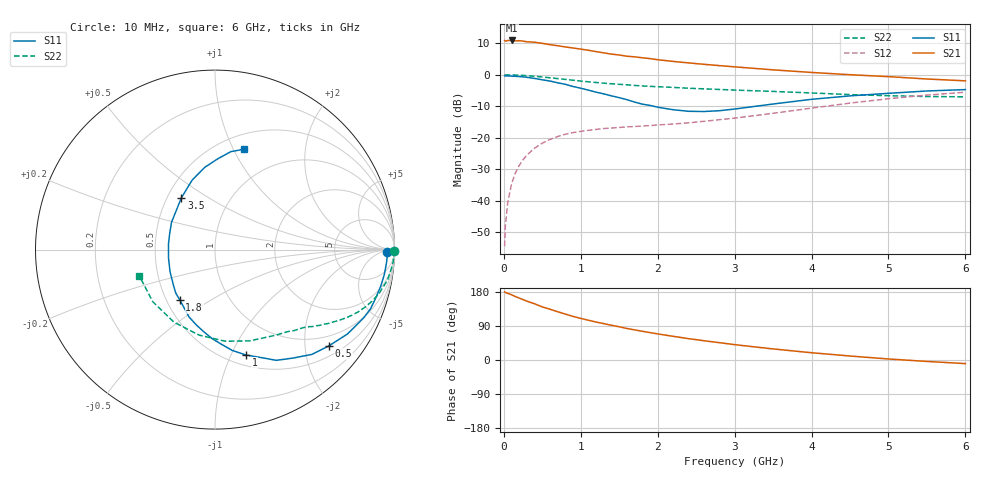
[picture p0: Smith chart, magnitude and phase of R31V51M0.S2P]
! SIEMENS Small Signal Semiconductors
! BFR181
! Si NPN RF Bipolar Junction Transistor in SOT23
! VCE = 1.5 V  IC = 1 mA
! Common Emitter S-Parameters:  May  1996
# GHz  S  MA  R  50
!  f  S11  S21  S12  S22
! GHz  MAG  ANG  MAG  ANG  MAG  ANG  MAG  ANG
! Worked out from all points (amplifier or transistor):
!   36 points, 10 MHz to 6 GHz, reference 50 ohm
!   highest |S21| = 10.9 dB at 100 MHz (marker M1)
!   |S21| within 3 dB of that: start of sweep to 1.068 GHz
!   unconditionally stable (mu >= 1): 1.968 GHz to 3.727 GHz
!   at 250 MHz: K = 0.16, MSG = 18.8 dB, |S12| = -27.0 dB
!   at 1.4 GHz: K = 0.78, MSG = 11.7 dB, |S12| = -16.9 dB
!   at 6 GHz: K = 0.89, MSG = 1.8 dB, |S12| = -5.5 dB
!   S11 on the Smith chart (normalised r, x): 10 MHz: 42, -16; 500 MHz: 0.73, -2.54; 1 GHz: 0.61, -1.14; 1.8 GHz: 0.59, -0.37; 3.5 GHz: 0.59, +0.39; 6 GHz: 0.65, +1.10
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0.01  0.9588 -0.9  3.478 179.5  0.0019 89.5  0.9987 -0.4
0.02  0.9605 -1.6  3.413 178.2  0.004 93.6  0.9934 -0.8
0.05  0.9586 -4.4  3.503 176.0  0.0092 87.2  0.997 -1.9
0.1  0.9534 -8.4  3.506 172.2  0.0185 84.1  0.9945 -4.0
0.15  0.9456 -12.5  3.454 167.3  0.0276 81.4  0.989 -5.9
0.2  0.9358 -16.5  3.476 163.4  0.0363 78.9  0.9825 -7.9
0.3  0.9111 -24.7  3.341 155.3  0.0533 74.4  0.9668 -11.4
0.4  0.8751 -32.5  3.288 148.3  0.0683 69.6  0.9466 -14.9
0.5  0.8304 -40.3  3.156 140.1  0.0821 65.1  0.9218 -18.1
0.7  0.7449 -54.2  2.894 127.4  0.1047 57.5  0.87 -23.5
0.9  0.651 -67.3  2.661 115.0  0.1207 51.6  0.8193 -27.8
1  0.6116 -73.7  2.555 109.7  0.1263 49.3  0.7943 -29.8
1.1  0.5699 -80.3  2.449 104.9  0.1314 47.4  0.773 -31.4
1.4  0.4623 -97.7  2.126 91.6  0.1428 43.5  0.72 -35.9
1.6  0.4022 -111.1  1.97 83.2  0.149 42.3  0.6932 -38.2
1.8  0.3417 -125.1  1.862 75.8  0.1538 42.6  0.6656 -40.5
2.2  0.2788 -154.1  1.63 62.5  0.165 43.7  0.6304 -45.7
2.8  0.2686 159.8  1.398 45.8  0.1934 47.8  0.585 -54.5
3.5  0.3436 123.1  1.197 29.2  0.2445 49.7  0.5442 -69.1
4.5  0.4623 97.0  1.002 10.5  0.3551 45.1  0.4846 -100.5
5.5  0.5528 80.8  0.857 -3.8  0.4757 32.6  0.4521 -140.1
6  0.5817 74.0  0.801 -9.5  0.5287 24.8  0.4462 -160.7
